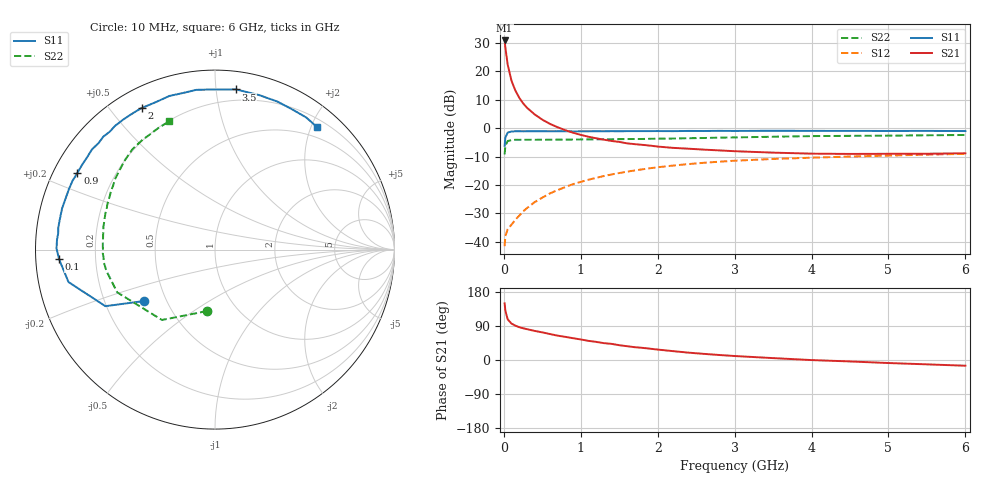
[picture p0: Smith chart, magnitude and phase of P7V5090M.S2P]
! SIEMENS Small Signal Semiconductors
! BFP196
! Si NPN RF Bipolar Junction Transistor in SOT143
! VCE = 0.5 V  IC = 90 mA
! Common Emitter S-Parameters:  May  1996
# GHz  S  MA  R  50
!  f  S11  S21  S12  S22
! GHz  MAG  ANG  MAG  ANG  MAG  ANG  MAG  ANG
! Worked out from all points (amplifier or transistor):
!   36 points, 10 MHz to 6 GHz, reference 50 ohm
!   highest |S21| = 30.8 dB at 10 MHz (marker M1)
!   |S21| within 3 dB of that: start of sweep to 22.31 MHz
!   unconditionally stable (mu >= 1): start of sweep to 15.48 MHz; 133.8 MHz to end of sweep
!   at 250 MHz: K = 1.24, MAG = 16.1 dB, |S12| = -29.3 dB
!   at 1.4 GHz: K = 1.27, MAG = 2.8 dB, |S12| = -16.3 dB
!   at 6 GHz: K = 1.08, MAG = -1.7 dB, |S12| = -9.0 dB
!   S11 on the Smith chart (normalised r, x): 10 MHz: 0.38, -0.28; 100 MHz: 0.07, -0.03; 900 MHz: 0.07, +0.26; 2 GHz: 0.08, +0.61; 3.5 GHz: 0.12, +1.13; 6 GHz: 0.32, +2.10
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0.01  0.4874 -144.0  34.85 149.5  0.0084 52.5  0.3451 -97.3
0.02  0.6871 -152.7  26.01 130.1  0.0127 41.8  0.491 -127.0
0.05  0.8359 -167.5  13.08 107.3  0.0167 35.2  0.5947 -156.4
0.1  0.8706 -176.5  6.766 96.0  0.0201 42.8  0.6165 -168.9
0.15  0.883 179.6  4.575 90.6  0.0246 49.2  0.6237 -173.6
0.2  0.8821 176.5  3.437 86.6  0.0289 53.8  0.6226 -176.2
0.25  0.8784 174.1  2.735 83.8  0.0342 57.1  0.6255 -178.1
0.3  0.8816 172.0  2.292 81.4  0.0392 59.5  0.624 -179.4
0.4  0.881 168.0  1.747 76.8  0.0499 62.3  0.6251 178.5
0.5  0.8824 164.9  1.41 72.9  0.06 63.9  0.6259 176.7
0.6  0.8797 161.0  1.188 68.5  0.0712 63.9  0.6261 175.2
0.7  0.881 157.4  1.036 64.2  0.0815 63.1  0.6273 173.8
0.9  0.8777 150.9  0.83 57.5  0.1036 61.0  0.6298 170.9
1.1  0.8787 144.2  0.705 50.5  0.1238 58.3  0.6349 168.3
1.6  0.8862 129.0  0.541 36.4  0.1716 49.9  0.643 161.7
2  0.8884 117.4  0.474 27.5  0.2051 42.5  0.6527 156.1
2.2  0.8853 111.9  0.45 23.4  0.2198 39.0  0.6567 153.5
2.8  0.8961 96.7  0.406 13.2  0.2571 28.8  0.681 145.0
3.5  0.9001 82.6  0.371 5.0  0.2872 17.7  0.7061 135.7
4.5  0.895 67.0  0.352 -3.8  0.3168 5.2  0.7322 124.0
5.5  0.8944 55.4  0.355 -11.5  0.3418 -5.6  0.7489 114.4
6  0.8887 50.1  0.361 -15.1  0.3532 -11.3  0.7579 109.6
